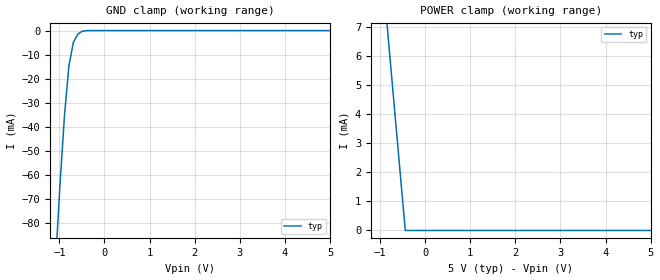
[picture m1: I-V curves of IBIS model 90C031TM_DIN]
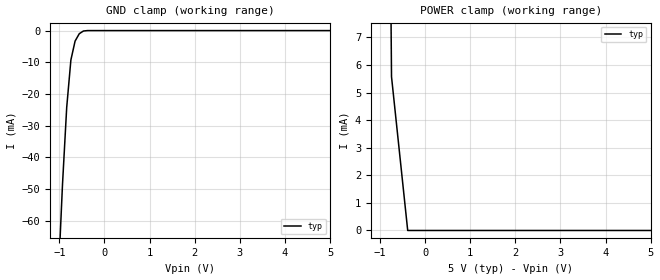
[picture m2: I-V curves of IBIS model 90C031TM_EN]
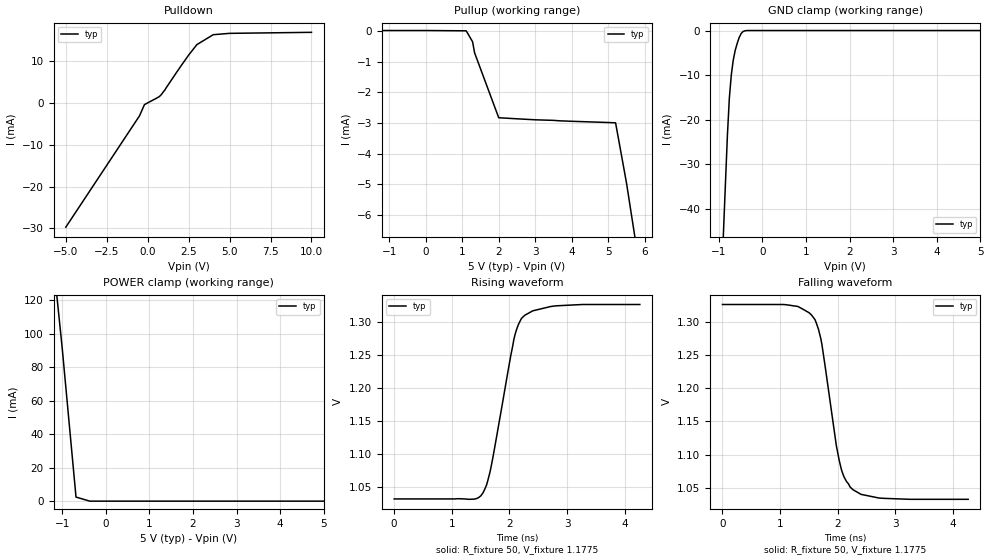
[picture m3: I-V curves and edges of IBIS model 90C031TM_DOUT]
|   National Semiconductor Corporation
|   Interface Products Group
|   IBIS Model of DS90C031TM
|   16L SOIC Package
[IBIS Ver]   3.2
[File name]   90c031tm.ibs
[File Rev]   2.1
[Date]   12/11/2002
[Source]   File originated at National Semiconductor Corporation.
   Data Transmission Products group. All data based on
   Empirical Measurements(Bench).
[Notes]   File created by SBH.
   See new data, ramp, rise, fall tables--milt
   Checked using ibischk3 ver 3.2.9
[Disclaimer]
(C) Copyright National Semiconductor Corporation 1994
   All rights reserved
   National Semiconductor Corporation hereby grants
the user of this IBIS model a non-exclusive, nontransferable
license to use this IBIS model under the following terms.
Before using this IBIS model, the user should read this
license.  If the user does not accept these terms,  the
IBIS model should be returned to National within 30 days.
   The user is granted this license only to use the
IBIS model and is not granted rights to sell, load, rent,
lease or license the IBIS model in whole or in part, or in
modified form to anyone other than user. User may modify
the IBIS model to suit its specific applications but rights
to derivative works and such modifications shall belong to
National.
   This IBIS model is provided on an "AS IS" basis and
National makes absolutely no warranty with respect to the
information contained herein.NATIONAL DISCLAIMS AND CUSTOMER
WAIVES ALL WARRANTIES, EXPRESS OR IMPLIED, INCLUDING
WARRANTIES OF MERCHANTABILITY OR FITNESS FOR A PARTICULAR
PURPOSE. The entire risk as to quality and performance is
with the Customer. ACCORDINGLY, IN NO EVENT SHALL THE
COMPANY BE LIABLE FOR ANY DAMAGES, WHETHER IN CONTRACT OR
TORT,INCLUDING ANY LOST PROFITS OR OTHER INCIDENTAL,
CONSEQUENTIAL, EXEMPLARY, OR PUNITIVE DAMAGES ARISING OUT
OF THE USE OR APPLICATION OF THE IBIS model provided in
this package.Further, National reserves the right to make
changes without notice to any product herein to improve
reliability, function, or design. National does not convey
any license under patent rights or any other intellectual
property rights, including those of third parties.
   National is not obligated to provide maintenance or support
for the licensed IBIS model.
Contact National at ATTN:INTERFACE APPLICATIONS/IBIS MODELS.
2900 Semiconductor Drive, M/S A2595, Santa Clara, CA 95052-8090
IBIS Open Forum disclaims all warranties. See DISCLAIM.TXT
in vhdl.org:/pub/IBIS/models for the full disclaimer.
[Copyright]   Copyright 1994, National Semiconductor, All Rights Reserved
[Component]   DS90C031TM
[Manufacturer]  National Semiconductor Corp
[Package]
|   typ   min   max
R_pkg   50.0m   NA   NA
L_pkg   1.37nH   NA   NA
C_pkg   0.1pF   NA   NA   |0.26pF
[Pin]   signal_name   model_name   R_pin   L_pin   C_pin
1   DIN1   90C031TM_DIN   50.0m   2.07n   0.429p
2   DOUT1+   90C031TM_DOUT   50.0m   1.49n   0.1p  |0.306p
3   DOUT1-   90C031TM_DOUT   50.0m   0.95n   0.1p |0.146p
4   EN   90C031TM_EN   50.0m   0.95n   0.152p
5   DOUT2-   90C031TM_DOUT   50.0m   0.95n   0.152p
6   DOUT2+   90C031TM_DOUT   50.0m   0.95n   0.146p
7   DIN2   90C031TM_DIN   50.0m   1.49n   0.306p
8   GND   GND   50.0m   2.07n   0.429p
9   DIN3   90C031TM_DIN   50.0m   2.07n   0.429p
10   DOUT3+   90C031TM_DOUT   50.0m   1.49n   0.306p
11   DOUT3-   90C031TM_DOUT   50.0m   0.95n   0.146p
12   EN*   90C031TM_EN   50.0m   0.95n   0.152p
13   DOUT4-   90C031TM_DOUT   50.0m   0.95n   0.152p
14   DOUT4+   90C031TM_DOUT   50.0m   0.95n   0.146p
15   DIN4   90C031TM_DIN   50.0m   1.49n   0.306p
16   VCC   POWER   50.0m   2.07n   0.429p
[Diff_pin]   inv_pin   vdiff   tdelay_typ   tdelay_min   tdelay_max
| The '+' pin is Diff_pin and the '-' pin is the inv_pin
2   3   NA   0 0 0
6   5   NA   0 0 0
10   11   NA   0 0 0
14   13   NA   0 0 0
| Models and submodels in the file (3): 90C031TM_DIN (Input), 90C031TM_EN (Input), 90C031TM_DOUT (3-state)
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|   Driver Input  MODEL
[Model]   90C031TM_DIN
Model_type   Input
|Signals   DIN1,DIN2,DIN3,DIN4
Vinh = 2.0
Vinl = 0.8
|   typ   min   max
C_comp   1.0pF   NA   NA
|   typ   min   max
[Temperature Range]   25.0   NA   NA
[Voltage range]   5.0V   4.5V   5.5V
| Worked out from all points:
|   GND clamp passes 1 mA (typ) near -0.55 V on its own axis
[Power_clamp]
| Note that the[POWER_clamp]voltage table is referenced to Vcc
| and is calculated using Vtable=Vcc - Vmeasured.
|   Voltage   I(typ)   I(min)   I(max)
-5V       80.3mA     NA         NA
-740mV    5.277mA    NA         NA
-437.9mV  140nA      NA         NA
5V        0A         NA         NA
[GND_clamp]
|   Voltage   I(typ)   I(min)   I(max)
-5V       -1.15A     NA         NA
-1.083V   -96.09mA   NA         NA
-984.2mV  -63.91mA   NA         NA
-885.8mV  -35.46mA   NA         NA
-787.4mV  -14.69mA   NA         NA
-688.9mV  -4.911mA   NA         NA
-590.5mV  -1.549mA   NA         NA
-492.1mV  -255.1uA   NA         NA
-393.7mV  0A         NA         NA
5V        0A         NA         NA
|   Driver Enable  MODEL
[Model]   90C031TM_EN
Model_type   Input
|Signals   EN,EN*
Vinh = 2.0
Vinl = 0.8
|   typ   min   max
C_comp   1.0pF   NA   NA
|   typ   min   max
[Temperature Range]   25.0   NA   NA
[Voltage range]   5.0V   4.5V   5.5V
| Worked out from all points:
|   GND clamp passes 1 mA (typ) near -0.56 V on its own axis
[GND_clamp]
|   Voltage   I(typ)   I(min)   I(max)
-5V       -1.33A     NA         NA
-1.022V   -77.96mA   NA         NA
-928.9mV  -48.51mA   NA         NA
-836.1mV  -24.26mA   NA         NA
-743.2mV  -9.271mA   NA         NA
-650.3mV  -3.324mA   NA         NA
-557.4mV  -993.2uA   NA         NA
-464.5mV  -130.4uA   NA         NA
5V        0A         NA         NA
[Power_clamp]
| Note that the[POWER_clamp]voltage table is referenced to Vcc
| and is calculated using Vtable=Vcc - Vmeasured.
|   Voltage   I(typ)   I(min)   I(max)
-5V       846mA      NA         NA
-743.2mV  5.575mA    NA         NA
-384.2mV  98.6nA     NA         NA
5V        0A         NA         NA
|   Driver Output  MODEL
[Model]   90C031TM_DOUT
Model_type   3-state
| Signals   DOUT1+,DOUT1-,DOUT2+,DOUT2-,DOUT3+,DOUT3-,DOUT4+,DOUT4-
Vmeas = 1.1775   |Reference voltage for timing measurements
Cref = 0.3pF   |Timing specification test load capacitance value
Rref = 50
Vref = 1.1775
| variable   typ   min   max
C_comp   0.01pF   NA   NA
|   typ   min   max
[Temperature Range]   25.0   NA   NA
[Voltage range]   5.0V   4.5V   5.5V
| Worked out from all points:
|   slope of the pulldown table from 0 to 0.75 V, typ, clamps not added: 456 ohm
|   GND clamp passes 1 mA (typ) near -0.51 V on its own axis
|   falling waveform, R_fixture 50, V_fixture 1.1775: 20-80 % time 303ps typ, NA min, NA max; typ from 1.33 V to 1.03 V
|   rising waveform, R_fixture 50, V_fixture 1.1775: 20-80 % time 360ps typ, NA min, NA max; typ from 1.03 V to 1.33 V
[Pulldown]
|new bench data as of 11/20/2003
|   Voltage   I(typ)   I(min)   I(max)
-5V       -29.7mA    NA         NA
-500mV    -3.105mA   NA         NA
-200mV    -436uA     NA         NA
800mV     1.828mA    NA         NA
1.03V     2.93mA     NA         NA
2.5V      11.4mA     NA         NA
3V        13.9mA     NA         NA
4V        16.28mA    NA         NA
5V        16.6mA     NA         NA
10V       16.84mA    NA         NA
[Pullup]
|new bench data as of 11/20/2003---milt
|   Voltage   I(typ)   I(min)   I(max)
| Note that the[Pullup]voltage table is referenced to Vcc
| and is calculated using Vtable=Vcc - Vmeasured.
-5V       10uA       NA         NA
1.11V     0A         NA         NA
1.284V    -357uA     NA         NA
1.34V     -719uA     NA         NA
2V        -2.83mA    NA         NA
5.2V      -2.995mA   NA         NA
5.5V      -4.962mA   NA         NA
10V       -39.4mA    NA         NA
[GND_clamp]
|   Voltage   I(typ)   I(min)   I(max)
| Outputs in Tri-state.
-5V       -1.04A     NA         NA
-850mV    -34.26mA   NA         NA
-805.3mV  -23.58mA   NA         NA
-760.5mV  -15.17mA   NA         NA
-715.8mV  -9.968mA   NA         NA
-671.1mV  -6.649mA   NA         NA
-626.3mV  -4.453mA   NA         NA
-536.8mV  -1.614mA   NA         NA
-492.1mV  -717.3uA   NA         NA
-447.4mV  -235.6uA   NA         NA
-313.2mV  0A         NA         NA
5V        0A         NA         NA
[POWER_clamp]
|   Voltage   I(typ)   I(min)   I(max)
| Note that the[POWER_clamp]voltage table is referenced to Vcc
| and is calculated using Vtable=Vcc - Vmeasured.
| Outputs in Tri-state.
-5V       1.11A      NA         NA
-1V       91.29mA    NA         NA
-684.2mV  2.428mA    NA         NA
-368.4mV  26.9nA     NA         NA
-52.63mV  0A         NA         NA
263.2mV   0A         NA         NA
5V        0A         NA         NA
[Ramp]
| Note: Ramp rate measured on single-ended Driver Output.
|   12/05/2002 at 12:10pm--milt
|   typ   min   max
dV/dt_r   0.176/360p   NA   NA
dV/dt_f   0.176/300p   NA   NA
R_load = 100Ohm | Note: This 100 Ohm is across the two driver output
| added Falling and Rising waveform measured on Tek scope TDS694C,probes=P6248
|  12/05/2002---milt
[Falling Waveform]
R_fixture=50
V_fixture=1.1775
V_fixture_min=1.29
V_fixture_max=1.29
0s        1.327V     NA         NA
1.304ns   1.324V     NA         NA
1.604ns   1.304V     NA         NA
1.724ns   1.266V     NA         NA
1.974ns   1.114V     NA         NA
2.024ns   1.091V     NA         NA
2.114ns   1.065V     NA         NA
2.264ns   1.047V     NA         NA
2.714ns   1.034V     NA         NA
4.26ns    1.033V     NA         NA
[Rising Waveform]
R_fixture=50
V_fixture=1.1775
V_fixture_min=1.29
V_fixture_max=1.29
0s        1.033V     NA         NA
1.304ns   1.032V     NA         NA
1.504ns   1.037V     NA         NA
1.604ns   1.054V     NA         NA
1.664ns   1.074V     NA         NA
2.094ns   1.28V      NA         NA
2.204ns   1.305V     NA         NA
2.264ns   1.31V      NA         NA
2.804ns   1.325V     NA         NA
4.26ns    1.327V     NA         NA
